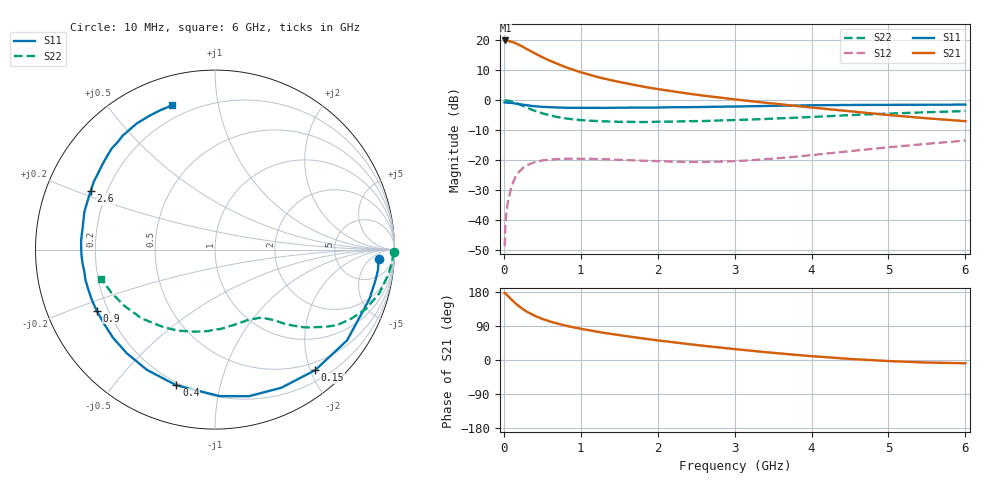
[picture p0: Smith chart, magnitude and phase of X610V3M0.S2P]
! SIEMENS Small Signal Semiconductors
! BFP193W
! Si NPN RF Bipolar Junction Transistor in SOT343
! VCE = 10 V  IC = 3 mA
! Common Emitter S-Parameters:  April 1994
# GHz  S  MA  R  50
!  f  S11  S21  S12  S22
! GHz  MAG  ANG  MAG  ANG  MAG  ANG  MAG  ANG
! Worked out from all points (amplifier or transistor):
!   40 points, 10 MHz to 6 GHz, reference 50 ohm
!   highest |S21| = 19.9 dB at 20 MHz (marker M1)
!   |S21| within 3 dB of that: start of sweep to 308 MHz
!   unconditionally stable (mu >= 1): 1.984 GHz to 4.647 GHz
!   at 200 MHz: K = 0.11, MSG = 21.2 dB, |S12| = -24.0 dB
!   at 1.5 GHz: K = 0.75, MSG = 13.0 dB, |S12| = -20.0 dB
!   at 6 GHz: K = 0.95, MSG = 3.2 dB, |S12| = -13.5 dB
!   S11 on the Smith chart (normalised r, x): 10 MHz: 15, -10; 150 MHz: 0.37, -2.08; 400 MHz: 0.19, -0.74; 900 MHz: 0.16, -0.24; 2.6 GHz: 0.14, +0.22; 6 GHz: 0.14, +0.74
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0.01  0.9133 -3.4  9.877 176.9  0.0036 84.9  0.9966 -0.8
0.02  0.9151 -7.0  9.916 175.7  0.0077 83.4  0.9893 -3.3
0.05  0.9034 -17.8  9.808 169.5  0.0188 79.9  0.9774 -7.8
0.1  0.8929 -34.5  9.448 159.3  0.0361 70.8  0.9473 -14.9
0.15  0.8735 -50.3  8.973 149.7  0.0514 62.9  0.9018 -21.7
0.2  0.8538 -64.4  8.345 141.3  0.0634 55.7  0.8489 -27.1
0.25  0.8384 -77.0  7.744 134.1  0.0739 49.4  0.7983 -31.9
0.3  0.817 -88.1  7.11 127.4  0.0811 44.2  0.7452 -35.3
0.4  0.7861 -105.9  6.066 116.9  0.0912 35.8  0.6622 -40.9
0.5  0.7699 -119.5  5.211 108.4  0.0976 29.9  0.6004 -44.7
0.6  0.7584 -130.5  4.534 101.7  0.1008 25.4  0.5533 -47.6
0.7  0.7509 -139.2  4.017 96.0  0.103 22.1  0.5184 -49.6
0.9  0.7417 -152.7  3.215 86.4  0.1046 17.4  0.4758 -53.6
1.1  0.7401 -162.3  2.683 78.8  0.104 14.5  0.4518 -57.3
1.3  0.7385 -170.8  2.29 71.8  0.1025 12.7  0.4404 -61.5
1.6  0.7456 179.4  1.894 62.7  0.0993 12.4  0.4316 -67.4
2.2  0.7577 163.7  1.396 46.9  0.0933 15.8  0.4356 -80.9
2.6  0.7655 154.7  1.183 37.4  0.0921 21.3  0.4454 -90.4
3.2  0.7869 142.8  0.961 24.8  0.0982 30.3  0.4719 -104.5
4.5  0.8271 121.8  0.649 2.8  0.1397 41.6  0.5598 -136.7
5.5  0.8341 111.4  0.495 -6.7  0.1852 40.4  0.625 -157.3
6  0.8388 106.5  0.443 -8.6  0.2102 38.5  0.6542 -165.6
